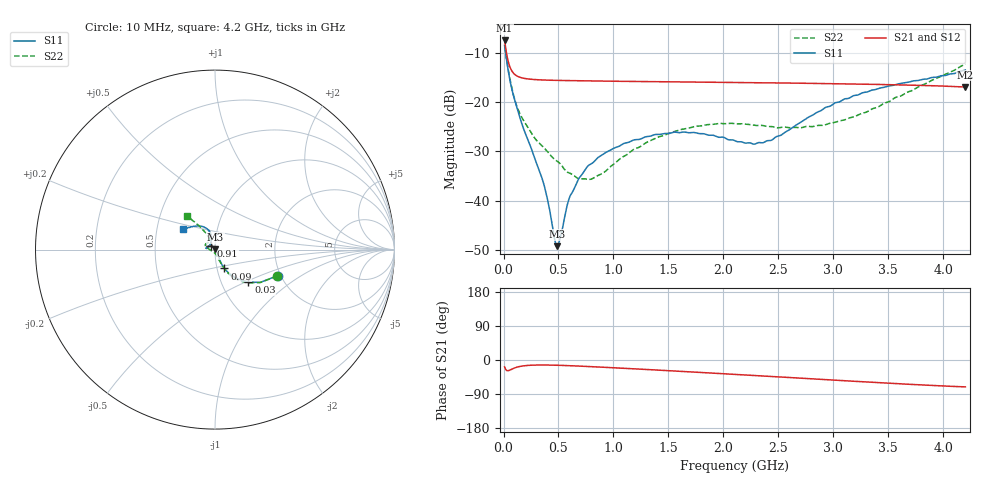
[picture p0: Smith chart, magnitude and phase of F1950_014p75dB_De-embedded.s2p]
! Integrated Device Technology
! Corporate Headquarters
! 6024 Silver Creek Valley Road
! San Jose, CA 95138  USA
! Phone:  1-408-284-8200
! Toll Free:  1-800-223-1366
! Webpage:  http://www.idt.com/
! Timing and RF Division
! 515 Groton Road, Suite 102
! Westford, MA 01886-6024
! Device:  F1950
! Description: 7-bit 0.25 dB Digital Step Attenuator
! Frequency:  150.0 -  4000.00 MHz
! Package:  4x4 mm Thin QFN Plastic Package: 24 pin
! Ports:  2 RF, 12 DC
!  Pin  1  = D0
!  Pin  2  = VDD
!  Pin  3  = Vmode
!  Pin  4  = GND
!  Pin  5  = RF1  =  Port 1
!  Pin  6  = GND
!  Pin  7  = GND
!  Pin  8  = GND
!  Pin  9  = GND
!  Pin 10  = GND
!  Pin 11  = GND
!  Pin 12  = GND
!  Pin 13  = GND
!  Pin 14  = RF2  =  Port 2
!  Pin 15  = GND
!  Pin 16  = LE
!  Pin 17  = CLK
!  Pin 18  = DATE
!  Pin 19  = D6
!  Pin 20  = D5
!  Pin 21  = D4
!  Pin 22  = D3
!  Pin 23  = D2
!  Pin 24  = D1
! State:  59
! Atten State:  14.75 dB
! Voltage:  +5.00 Volts
! Current:  Not Measured mA
! Data:  The device was measured on a the F195X evaluation board which has
!  individual transmission lines to the RF pins.  Data was collected
!  using a calibrated network analyzer.  The evaluation board was
!  de-embedded using a TRL calibration technique.
!  The reference plane is the edge of the package pin.
! Misc:  Board 2019
!  Action Tracker AT0250
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# GHz S dB R 50
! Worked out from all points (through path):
!   420 points, 10 MHz to 4.2 GHz, reference 50 ohm
!   highest |S21| = -7.44 dB at 10 MHz (marker M1); lowest = -16.9 dB at 4.2 GHz (marker M2)
!   group delay of S21, straight-line fit = 41.2 ps
!   lowest |S11| = -49.3 dB at 490 MHz (marker M3), VSWR 1.01, Z = 50.2 + j0.25 ohm
!   |S11| at or under -10 dB: 19.28 MHz to end of sweep
!   |S22| runs from -35.7 to -8.5 dB; largest |S21 - S12| = 0.00023
!   S11 on the Smith chart (normalised r, x): 10 MHz: 1.93, -0.65; 30 MHz: 1.34, -0.52; 90 MHz: 1.08, -0.23; 910 MHz: 0.95, +0.04; 4.2 GHz: 0.68, +0.16
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0.01  -8.43 -22.4  -7.44 -18.2  -7.44 -18.2  -8.46 -22.9
0.03  -11.71 -44.2  -10.37 -27.8  -10.37 -27.8  -11.62 -45.0
0.05  -14.52 -54.6  -12.29 -27.6  -12.29 -27.6  -14.29 -55.6
0.09  -18.61 -63.6  -14.08 -22.3  -14.08 -22.3  -18.46 -63.1
0.18  -25.24 -63.7  -15.11 -15.5  -15.11 -15.5  -23.63 -68.9
0.36  -36.17 -47.4  -15.48 -13.2  -15.48 -13.2  -29.07 -73.8
0.41  -40.82 -38.2  -15.52 -13.3  -15.52 -13.4  -30.30 -74.5
0.46  -47.29 -4.9  -15.55 -13.6  -15.55 -13.7  -31.54 -79.7
0.49  -49.27 46.4  -15.56 -13.9  -15.56 -13.9  -32.03 -82.9
0.52  -47.17 84.7  -15.58 -14.1  -15.57 -14.2  -32.62 -84.1
0.6  -39.38 116.8  -15.61 -15.0  -15.61 -15.0  -34.42 -96.7
0.71  -34.78 128.5  -15.64 -16.3  -15.64 -16.4  -35.57 -116.2
0.91  -30.52 141.8  -15.70 -19.1  -15.70 -19.2  -34.33 -156.6
1.17  -27.79 154.9  -15.77 -23.0  -15.77 -23.0  -29.79 177.8
1.41  -26.54 165.5  -15.83 -26.8  -15.83 -26.8  -27.05 167.8
1.73  -26.14 172.5  -15.90 -31.8  -15.90 -31.8  -24.97 158.9
2.11  -27.89 163.0  -15.99 -38.1  -15.99 -38.2  -24.38 149.3
2.43  -27.77 128.5  -16.07 -43.3  -16.07 -43.3  -24.94 139.3
2.81  -22.63 105.7  -16.17 -49.8  -16.16 -49.8  -24.95 123.9
3.1  -19.34 107.6  -16.26 -54.7  -16.25 -54.7  -23.59 118.3
3.51  -16.67 118.5  -16.42 -61.3  -16.42 -61.4  -19.83 118.6
4.2  -13.45 147.3  -16.91 -70.9  -16.90 -71.0  -12.24 129.6
